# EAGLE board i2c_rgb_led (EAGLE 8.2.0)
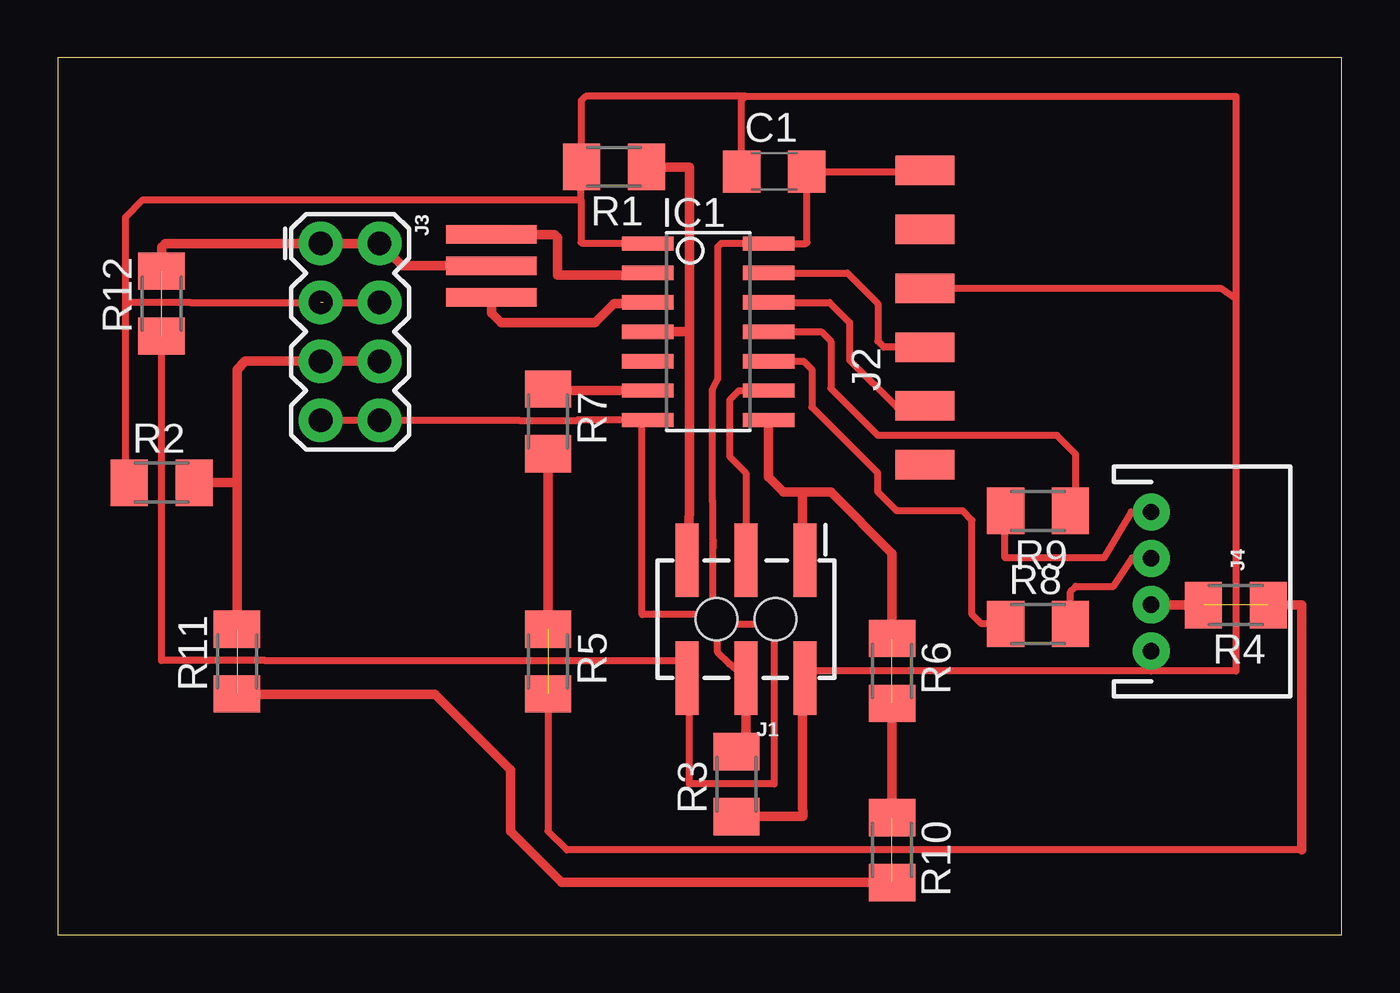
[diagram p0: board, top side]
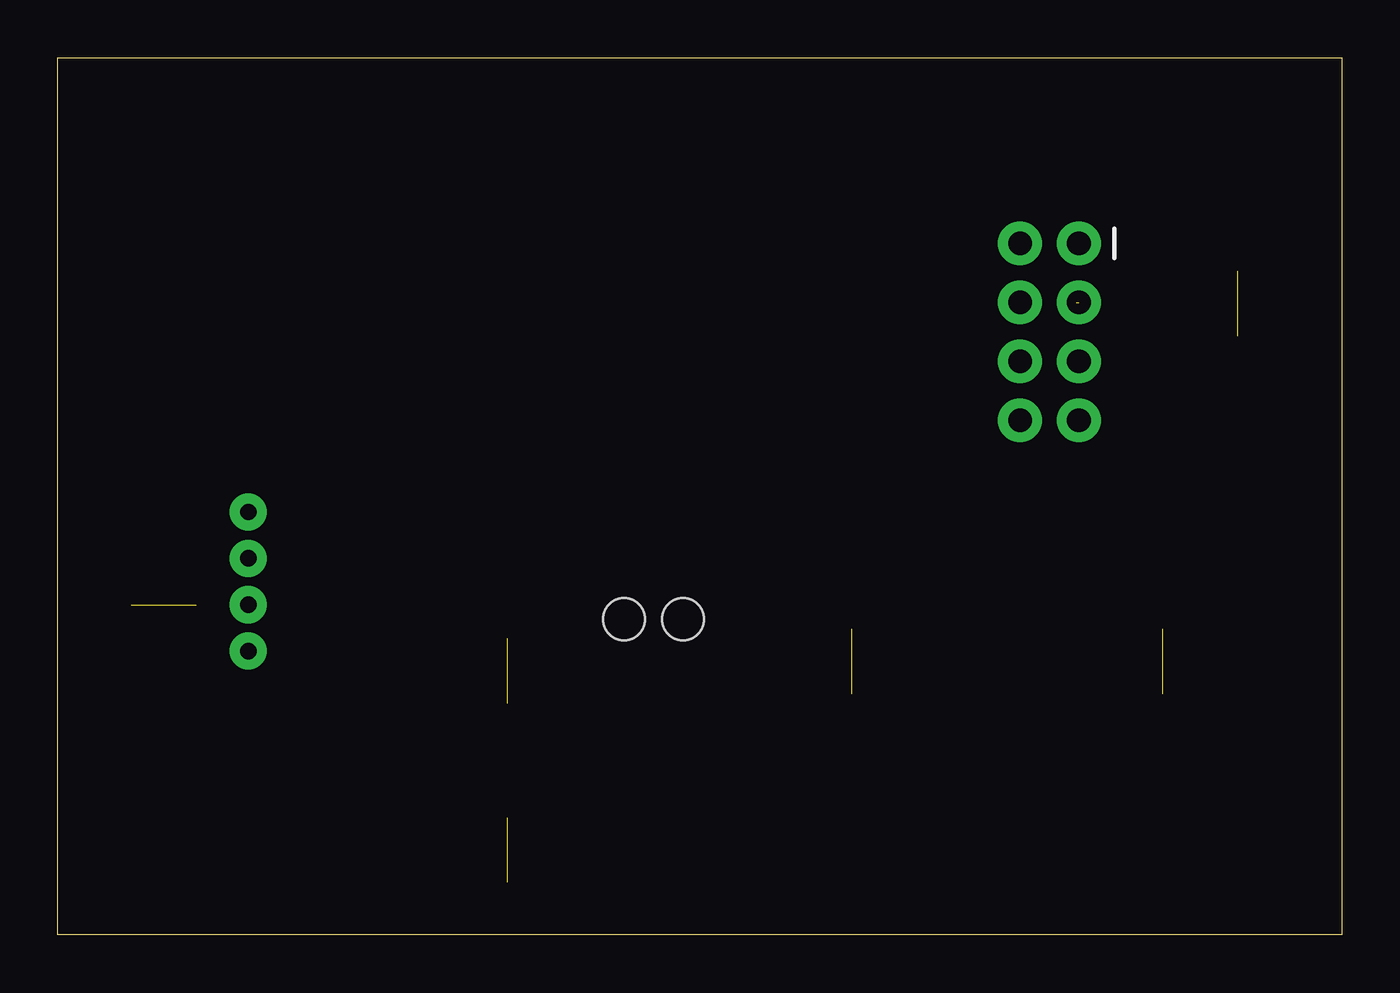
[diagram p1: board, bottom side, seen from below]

Size 55.35 x 37.82 mm. Coordinates in mm from the lower left corner, seen from the top.
Outline: 0,0 55.35,0 55.35,37.82 0,37.82 0,0
Copper layers (1*16): Top 0.035mm / dielectric 1.5mm / Bottom 0.035mm
Design rules "default *": minimum track width 6mil, minimum drill 0.35mm, track to track 16mil, track to pad 16mil, pad to pad 16mil, via to via 16mil, smd to smd 16mil, copper to edge 40mil, drill to drill 6mil, minimum pad ring 10mil, minimum via ring 8mil, stop-mask expansion 4mil, vias tented up to drill 0mil, thermal gap 10mil

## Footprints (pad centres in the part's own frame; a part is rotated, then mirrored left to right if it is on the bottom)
C1206 = smd 1.6 x 1.8: 1 -1.4,0; 2 1.4,0
SOIC14 = smd 0.61 x 2.21: 1 -3.81,-2.603; 2 -2.54,-2.603; 3 -1.27,-2.603; 4 0,-2.603; 5 1.27,-2.603; 6 2.54,-2.603; 7 3.81,-2.603; 8 3.81,2.603; 9 2.54,2.603; 10 1.27,2.603; 11 0,2.603; 12 -1.27,2.603; 13 -2.54,2.603; 14 -3.81,2.603
2X3_SMT_POSTS = smd 1 x 3.17: 1 -2.54,-2.54; 2 -2.54,2.54; 3 0,-2.54; 4 0,2.54; 5 2.54,-2.54; 6 2.54,2.54 | hole 1.8: -1.27,0; 1.27,0
1X06SMD = smd 2.54 x 1.27: 1 0,6.35; 2 0,3.81; 3 0,1.27; 4 0,-1.27; 5 0,-3.81; 6 0,-6.35
2X4 = drill 1.016 pad 1.88: 1 -3.81,-1.27; 2 -3.81,1.27; 3 -1.27,-1.27; 4 -1.27,1.27; 5 1.27,-1.27; 6 1.27,1.27; 7 3.81,-1.27; 8 3.81,1.27
JST-4-PTH = drill 0.7 pad 1.6: 1 -3,0; 2 -1,0; 3 1,0; 4 3,0
M1206 = smd 1.6 x 2: 1 -1.4,0; 2 1.4,0
EFOBM = smd 0.8 x 3.9: 1 -1.35,0; 2 0,0; 3 1.35,0

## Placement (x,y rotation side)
C1  1uF  [C1206]  30.89,32.92 0 top
IC1  ATTINY44-SSU  [SOIC14]  28.04,26.01 270 top
J1  [2X3_SMT_POSTS]  29.67,13.61 180 top
J2  FTDI-SMD-HEADER  [1X06SMD]  37.39,26.62 0 top
J3  [2X4]  12.6,26.01 270 top
J4  [JST-4-PTH]  47.14,15.24 270 top
R1  10k  [M1206]  23.98,33.12 180 top
R2  4.9k  [M1206]  4.47,19.51 0 top
R3  4.9k  [M1206]  29.26,6.5 90 top
R4  0  [M1206]  50.8,14.22 180 top
R5  0  [M1206]  21.13,11.79 270 top
R6  0  [M1206]  35.97,11.38 270 top
R7  500  [M1206]  21.13,22.15 270 top
R8  1k  [M1206]  42.27,13.41 0 top
R9  1k  [M1206]  42.27,18.29 180 top
R10  0  [M1206]  35.97,3.66 270 top
R11  0  [M1206]  7.72,11.79 90 top
R12  0  [M1206]  4.47,27.23 90 top
XTAL1  20MHZ  [EFOBM]  18.69,28.85 270 top

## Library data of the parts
C1 R1-R12 = rcl
IC1 J2 XTAL1 = fab
J1 = SparkFun-Connectors; PROD_ID: CONN-11415
J3 = SparkFun-Connectors
J4 = SparkFun-Connectors; PROD_ID: WIRE-13531; SF_ID: PRT-09916

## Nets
CTS: J2.2
GND: C1.2 IC1.14 J1.6 J2.1 J3.1 J3.2 R12.1 R12.2 XTAL1.2
MISO: IC1.8 J1.1 J3.5 J3.6 R2.2 R6.1 R6.2 R10.1 R10.2 R11.1 R11.2
MOSI: IC1.7 J1.4 J3.7 J3.8 R3.2
RGB_B: J4.3 R4.1 R4.2 R5.1 R5.2 R7.2
RGB_G: J4.2 R8.2
RGB_R: J4.1 R9.2
RST: IC1.4 J1.5 R1.1
RTS: J2.6
RXD: IC1.12 J2.5
SCK: IC1.9 J1.3
TO_RGB_B: IC1.6 R7.1
TO_RGB_G: IC1.10 R8.1
TO_RGB_R: IC1.11 R9.1
TXD: IC1.13 J2.4
VCC: C1.1 IC1.1 J1.2 J2.3 J3.3 J3.4 J4.4 R1.2 R2.1 R3.1
XTAL1: IC1.2 XTAL1.1
XTAL3: IC1.3 XTAL1.3

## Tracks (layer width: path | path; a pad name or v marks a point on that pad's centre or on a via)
GND  (1 unrouted)
  Top 0.305: 32.51,32.92 37.34,32.92 | 27.23,11.58 27.23,6.5 30.89,6.5 30.89,13.41 29.26,13.41 28.24,14.43 28.24,16.66 | 32.31,32.71 32.31,29.87 32.26,29.82 IC1.14 28.6,29.82 28.45,29.67 28.45,23.99 28.23,23.56 28.23,18.69 | R12.1 4.47,11.83 6.49,11.83 8.93,11.83 27.19,11.83 27.23,11.79 | 28.23,18.67 28.23,18.69 | 28.24,16.66 28.24,16.91 | 28.24,17.04 28.24,16.66 | 28.24,17.04 28.24,17.05 | 28.23,18.69 28.23,17.05 28.24,17.04
  Top 0.406: 27.23,11.79 J1.6 27.23,11.58 | C1.2 32.51,32.92 32.31,32.71 | 37.34,32.92 J2.1 | 30.49,29.87 IC1.14 | XTAL1.2 14.83,28.85 J3.2 J3.1 4.62,29.82 4.47,29.67 R12.2
MISO  (3 unrouted)
  Top 0.406: R11.2 7.72,19.51 | 7.72,19.51 R2.2 | 7.72,19.51 7.72,24.38 8.08,24.74 J3.5 J3.6 | 32.11,19.1 31.29,19.1 30.65,19.75 IC1.8 | 32.11,19.1 32.11,16.26 J1.1 | 32.11,19.1 33.32,19.1 35.97,16.46 R6.1 | R6.2 R10.1 | R10.2 21.72,2.26 19.51,4.47 19.51,7.11 16.26,10.36 7.74,10.36 R11.1
MOSI
  Top 0.305: J1.4 28.96,11.68 28.45,12.19 28.45,13 27.64,13.82 25.2,13.82 25.2,22.2 | J3.7 J3.8 19.89,22.2 19.9,22.19 22.36,22.19 22.37,22.2 25.2,22.2 | 25.2,22.2 IC1.7
  Top 0.406: J1.4 29.67,8.71 R3.2
RGB_B  (2 unrouted)
  Top 0.305: R5.2 21.13,4.47 21.95,3.66 53.64,3.66
  Top 0.406: J4.3 48.98,14.24 R4.2 | R7.2 R5.1 | R4.1 53.64,14.22 53.64,3.66
RGB_G
  Top 0.305: R8.2 43.67,14.81 43.89,15.04 45.52,15.04 46.33,16.26 47.13,16.26 J4.2
RGB_R
  Top 0.305: J4.1 46.28,18.24 45.11,16.26 40.84,16.26 40.84,18.27
  Top 0.406: 40.84,18.27 R9.2
RST
  Top 0.406: IC1.4 27.23,26.01 | 27.23,26.01 27.23,23.16 27.23,18.29 J1.5 | 27.23,26.01 27.23,33.12 R1.1
RXD
  Top 0.305: IC1.12 33.27,27.28 34.14,26.42 34.14,24.79 36.17,22.76 37.34,22.76 J2.5
SCK
  Top 0.305: IC1.9 29.36,23.47 28.98,23.09 28.98,20.6 29.67,19.91 J1.3
TO_RGB_B
  Top 0.406: IC1.6 21.21,23.47 R7.1
TO_RGB_G
  Top 0.305: R8.1 39.83,13.41 39.42,13.82 39.42,17.88 39.01,18.29 36.17,18.29 35.36,19.1 35.36,19.91 32.51,22.76 32.51,24.38 32.16,24.74 IC1.10
TO_RGB_R
  Top 0.305: 43.89,18.51 43.89,20.73 43.08,21.54 35.36,21.54 33.32,23.57 33.32,25.6 32.92,26.01 IC1.11
  Top 0.406: 43.89,18.51 R9.1
TXD
  Top 0.305: J2.4 35.61,25.35 35.36,25.6 35.36,27.23 34.04,28.55 IC1.13
  Top 0.406: 30.75,28.45 IC1.13
VCC  (1 unrouted)
  Top 0.305: IC1.1 22.61,29.82 22.56,29.87 22.56,31.7 | 22.56,31.7 22.56,33.1 | 47.14,11.38 50.8,11.38 50.8,27.43 | J2.3 50.14,27.89 50.8,27.43 | R1.2 22.58,35.99 22.76,36.17 29.67,36.17 | 29.67,36.17 50.8,36.17 50.8,27.43 | C1.1 29.49,35.99 29.67,36.17 | 47.14,11.38 J4.4 | 3.09,27.27 3.05,27.23 | 3.09,27.27 5.7,27.27 5.71,27.28 11.43,27.28 J3.4 | R2.1 2.91,19.67 2.91,27.09 | 3.09,27.27 2.91,27.09 | 2.91,27.09 2.91,30.95 3.66,31.7 22.56,31.7 | J1.2 32.51,11.38 47.14,11.38
  Top 0.406: 22.56,33.1 R1.2 | R3.1 32.13,5.1 32.11,5.69 32.11,10.97 J1.2
XTAL1
  Top 0.406: XTAL1.1 21.41,30.2 21.54,30.07 21.54,28.45 25.34,28.45 IC1.2
XTAL3
  Top 0.406: XTAL1.3 18.69,26.82 19.1,26.42 23.16,26.42 23.98,27.23 25.39,27.23 IC1.3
